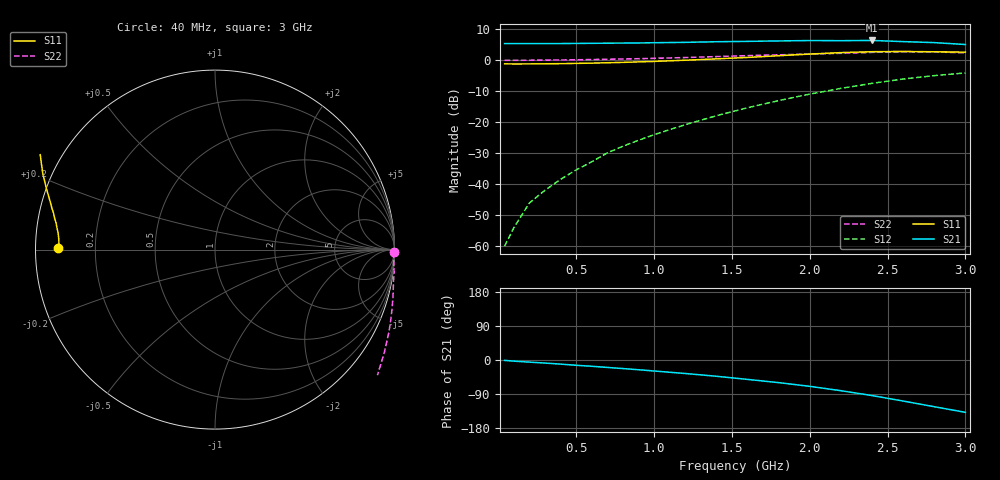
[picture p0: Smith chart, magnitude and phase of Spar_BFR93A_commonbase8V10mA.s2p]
! Filename:  BFR93ACF.S2P  Version:  2.0
! NXP part #: BFR93A  Date: Jul 1990
! Bias condition: Vce=8V, Ic=10mA
! COMMON BASE
#  MHz  S  MA  R  50
! Freq  S11  S21  S12  S22
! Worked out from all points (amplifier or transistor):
!   21 points, 40 MHz to 3 GHz, reference 50 ohm
!   highest |S21| = 6.4 dB at 2.4 GHz (marker M1)
!   |S21| within 3 dB of that: start of sweep to end of sweep
!   unconditionally stable (mu >= 1): start of sweep to 43.04 MHz
!   at 300 MHz: K = -0.60, MSG = 23.7 dB, |S12| = -41.9 dB
!   at 1 GHz: K = -0.92, MSG = 14.8 dB, |S12| = -24.0 dB
!   at 3 GHz: K = -0.72, MSG = 4.6 dB, |S12| = -4.1 dB
40  0.872 179.3  1.854 -1.0  0.001 50.9  0.996 -0.8
100  0.87 178.1  1.853 -3.0  0.002 81.4  0.995 -2.5
200  0.871 176.7  1.856 -5.6  0.005 105.3  0.999 -4.7
300  0.875 175.2  1.855 -8.1  0.008 122.1  1.006 -7.1
400  0.88 173.7  1.856 -10.9  0.012 127.9  1.009 -9.6
500  0.888 172.3  1.865 -13.9  0.017 133.7  1.016 -12.1
600  0.897 170.6  1.872 -16.6  0.023 136.7  1.025 -14.6
700  0.91 169.0  1.881 -19.6  0.032 138.8  1.035 -17.3
800  0.922 167.3  1.888 -22.6  0.041 141.0  1.046 -19.9
900  0.939 165.6  1.898 -25.7  0.051 141.9  1.058 -22.5
1000  0.956 163.8  1.914 -29.0  0.063 142.1  1.072 -25.3
1200  0.999 160.1  1.941 -35.6  0.091 141.9  1.104 -31.3
1400  1.051 156.0  1.985 -42.9  0.127 139.7  1.144 -37.7
1600  1.108 151.5  2.012 -51.2  0.171 137.3  1.184 -44.6
1800  1.181 146.1  2.046 -59.7  0.223 133.0  1.221 -52.5
2000  1.255 140.3  2.074 -69.5  0.284 127.8  1.257 -61.5
2200  1.326 134.2  2.065 -81.0  0.351 121.7  1.292 -72.2
2400  1.371 126.7  2.082 -93.8  0.423 114.1  1.338 -83.7
2600  1.383 118.2  1.995 -108.3  0.497 106.0  1.366 -95.2
2800  1.367 108.4  1.922 -123.3  0.564 96.9  1.361 -106.8
3000  1.348 98.6  1.791 -138.1  0.623 89.2  1.312 -118.1
